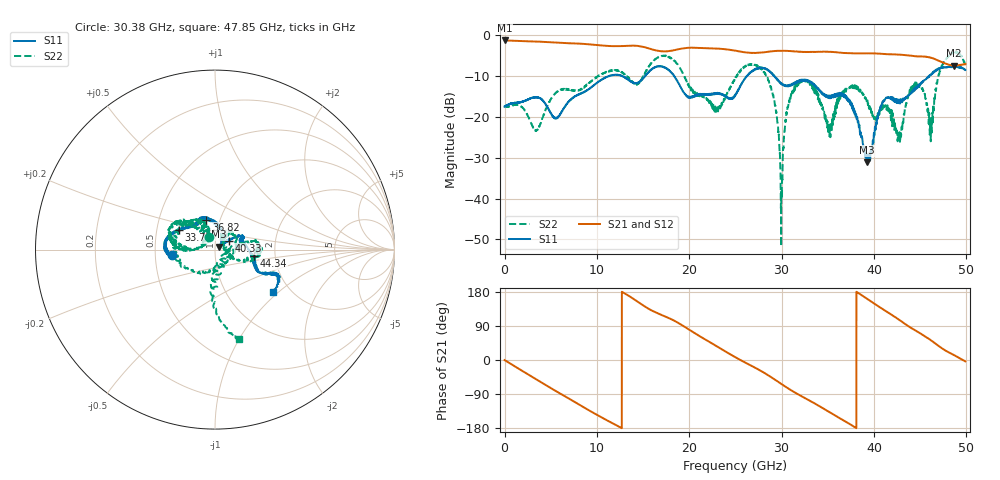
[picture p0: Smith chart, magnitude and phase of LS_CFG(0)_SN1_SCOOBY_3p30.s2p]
!Keysight Technologies,N5245B,MY58422026,A.13.80.08
!Date: Thursday, March 19, 2020 23:26:36
!Correction: S11(Full 2 Port(1,2))
!S21(Full 2 Port(1,2))
!S12(Full 2 Port(1,2))
!S22(Full 2 Port(1,2))
!S2P File: Measurements: S11, S21, S12, S22:
# Hz S DB R 50.0
!freq dBS11 angS11 dBS21 angS21 dBS12 angS12 dBS22 angS22
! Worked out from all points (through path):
!   4991 points, 10 MHz to 49.91 GHz, reference 50 ohm
!   highest |S21| = -1.35 dB at 20 MHz (marker M1); lowest = -7.5 dB at 48.67 GHz (marker M2)
!   group delay of S21, straight-line fit = 39.9 ps
!   lowest |S11| = -31.1 dB at 39.21 GHz (marker M3), VSWR 1.06, Z = 52.3 + j1.62 ohm
!   |S11| at or under -10 dB: start of sweep to 11.36 GHz; 18.37 GHz to 26.29 GHz (7.918 GHz wide, 35.5 % of centre); 29.22 GHz to 46.02 GHz (16.8 GHz wide, 44.7 % of centre)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
!   |S22| runs from -51.6 to -4.1 dB; largest |S21 - S12| = 0.0078
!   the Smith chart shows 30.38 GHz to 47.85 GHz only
!   S11 on the Smith chart (normalised r, x): 30.38 GHz: 0.61, -0.04; 33.73 GHz: 0.65, +0.15; 36.82 GHz: 0.86, +0.30; 40.33 GHz: 1.16, +0.11; 44.34 GHz: 1.55, -0.12; 47.85 GHz: 1.63, -0.93
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1e7  -17.54 -1.4  -1.35 -0.3  -1.34 -0.3  -17.16 0.7
2e7  -17.43 -0.7  -1.35 -0.4  -1.34 -0.4  -17.30 -0.5
8.33e9  -14.31 -65.4  -2.16 -121.2  -2.16 -121.2  -13.20 -67.8
1.665e10  -7.69 -129.7  -3.89 122.4  -3.88 122.4  -5.45 -163.0
2.289e10  -14.47 -136.4  -3.33 37.6  -3.33 37.7  -18.81 166.7
2.496e10  -14.90 -116.7  -3.82 7.8  -3.81 7.9  -10.77 -177.1
2.839e10  -8.38 -163.3  -4.17 -37.8  -4.16 -37.7  -10.02 -89.1
2.998e10  -12.05 -174.1  -3.88 -63.2  -3.88 -63.1  -38.55 1.0
3.038e10  -12.37 -173.1  -3.90 -69.7  -3.89 -69.6  -22.10 113.3
3.328e10  -11.59 159.7  -4.16 -110.6  -4.15 -110.3  -12.30 171.5
3.373e10  -12.80 151.9  -4.16 -116.5  -4.14 -116.2  -13.53 172.9
3.518e10  -15.10 124.9  -4.11 -137.4  -4.05 -137.1  -24.77 137.8
3.682e10  -15.18 106.1  -4.42 -161.0  -4.31 -161.1  -13.76 129.0
3.921e10  -31.13 33.8  -4.49 162.3  -4.47 162.0  -16.24 -125.5
4.033e10  -20.93 32.0  -4.54 144.1  -4.54 143.8  -20.02 -22.5
4.16e10  -15.17 26.1  -4.72 124.3  -4.74 124.1  -18.19 57.7
4.275e10  -15.88 17.1  -4.82 105.7  -4.85 105.5  -24.40 11.5
4.434e10  -13.18 -9.7  -5.17 80.0  -5.19 79.8  -12.00 -5.5
4.616e10  -9.69 -24.0  -5.55 52.2  -5.56 52.1  -26.00 -42.4
4.785e10  -7.90 -36.4  -7.09 23.4  -7.11 23.3  -5.75 -75.2
4.867e10  -7.53 -52.3  -7.49 13.0  -7.50 13.0  -4.12 -57.6
4.991e10  -8.58 -52.0  -7.13 -3.7  -7.15 -3.9  -7.33 -28.4
